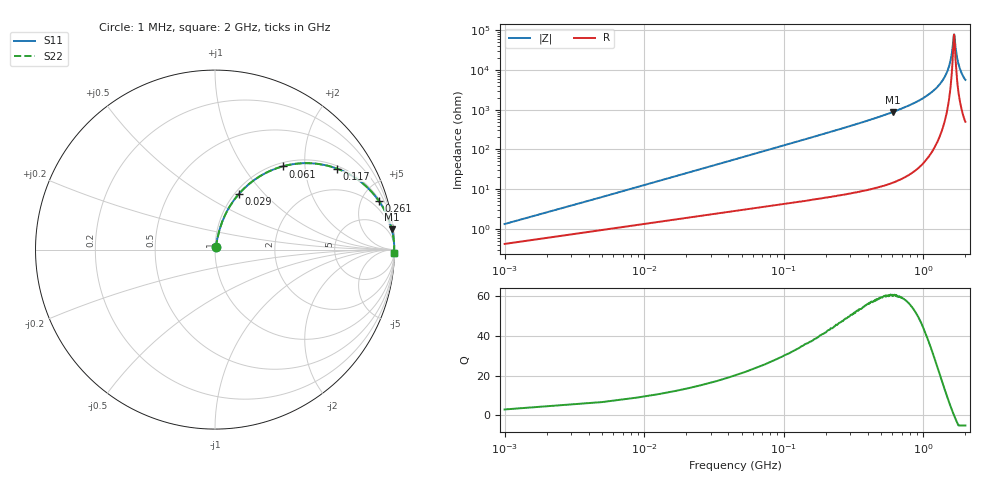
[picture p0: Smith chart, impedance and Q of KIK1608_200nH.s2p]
!version-2
!date-01.2022
!Series
# MHz S RI R 50
!Freq ReS11 ImS11 ReS21 ImS21 ReS12 ImS12 ReS22 ImS22
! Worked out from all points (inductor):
!   501 points, 1 MHz to 2 GHz, reference 50 ohm
!   read as one part in series: L = 200 nH near 9 MHz
!   highest Q = 60.3 at 601 MHz (marker M1), where L = 230 nH
!   self-resonance near 1.657 GHz
!   S11 on the Smith chart (normalised r, x): 1 MHz: 1.01, +0.03; 29 MHz: 1.05, +0.73; 61 MHz: 1.07, +1.54; 117 MHz: 1.09, +2.96; 261 MHz: 1.14, +6.73; 2 GHz: open
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1  0.00433 0.0125  0.9957 -0.0125  0.9957 -0.0125  0.00433 0.0125
13  0.0398 0.1545  0.9603 -0.1545  0.9603 -0.1545  0.0398 0.1545
21  0.0805 0.2381  0.9195 -0.2381  0.9195 -0.2381  0.0805 0.2381
29  0.1323 0.3093  0.8677 -0.3093  0.8677 -0.3093  0.1323 0.3093
61  0.3763 0.4636  0.6237 -0.4636  0.6237 -0.4636  0.3763 0.4636
117  0.6809 0.4509  0.3191 -0.4509  0.3191 -0.4509  0.6809 0.4509
177  0.8289 0.3641  0.1711 -0.3641  0.1711 -0.3641  0.8289 0.3641
261  0.914 0.27  0.086 -0.27  0.086 -0.27  0.914 0.27
337  0.9476 0.2136  0.0524 -0.2136  0.0524 -0.2136  0.9476 0.2136
601  0.9851 0.1132  0.0149 -0.1132  0.0149 -0.1132  0.9851 0.1132
669  0.9885 0.0984  0.0115 -0.0984  0.0115 -0.0984  0.9885 0.0984
1003  0.9963 0.05  0.00367 -0.05  0.00367 -0.05  0.9963 0.05
1337  0.9985 0.0207  0.00154 -0.0207  0.00154 -0.0207  0.9985 0.0207
1450  0.9987 0.013  0.00132 -0.013  0.00132 -0.013  0.9987 0.013
1530  0.9987 0.00783  0.00125 -0.00783  0.00125 -0.00783  0.9987 0.00783
1590  0.9988 0.00416  0.00124 -0.00416  0.00124 -0.00416  0.9988 0.00416
1653  0.9987 0.000405  0.00127 -0.000405  0.00127 -0.000405  0.9987 0.000405
1670  0.9987 -0.000511  0.00128 0.000511  0.00128 0.000511  0.9987 -0.000511
1720  0.9987 -0.00343  0.00133 0.00343  0.00133 0.00343  0.9987 -0.00343
1780  0.9986 -0.00669  0.00141 0.00669  0.00141 0.00669  0.9986 -0.00669
1880  0.9984 -0.0119  0.0016 0.0119  0.0016 0.0119  0.9984 -0.0119
2000  0.9981 -0.0176  0.00188 0.0176  0.00188 0.0176  0.9981 -0.0176
